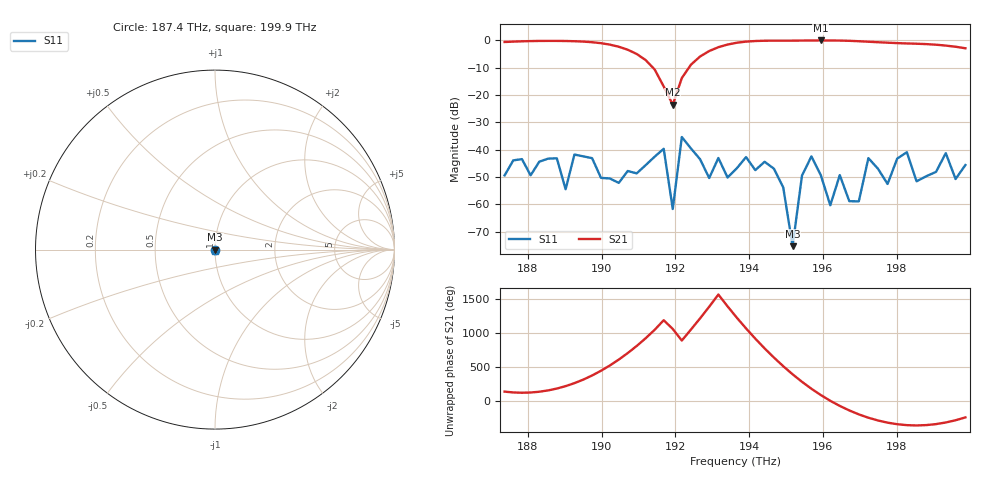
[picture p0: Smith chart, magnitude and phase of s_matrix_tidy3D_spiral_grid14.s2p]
[Version] 2.0
# Hz S RI
[Number of Ports] 2
[Two-Port Data Order] 12_21
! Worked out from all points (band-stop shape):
!   51 points, 187.4 THz to 199.9 THz, reference 50 ohm
!   highest |S21| = -0.05 dB at 195.9 THz (marker M1); lowest = -23.5 dB at 191.9 THz (marker M2)
!   |S21| within 3 dB of the highest: start of sweep to 190.6 THz; 193.1 THz to end of sweep
!   lowest |S11| = -75.3 dB at 195.2 THz (marker M3), VSWR 1.00, Z = 50 + j0.0138 ohm
!   |S11| at or under -10 dB: start of sweep to end of sweep
!   S12 and S22 are empty: the file has one direction only
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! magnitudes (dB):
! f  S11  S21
! 187.4 THz  -49.4  -0.6
! 188.8 THz  -43.1  -0.2
! 189 THz  -54.5  -0.3
! 189.5 THz  -42.4  -0.5
! 190.5 THz  -52.1  -2.3
! 191.7 THz  -39.7  -16.9
! 191.9 THz  -61.7  -23.5
! 192.2 THz  -35.4  -13.8
! 192.9 THz  -50.4  -3.9
! 193.7 THz  -46.8  -0.9
! 194.7 THz  -46.9  -0.1
! 195.2 THz  -75.3  -0.1
! 195.4 THz  -49.5  -0.1
! 195.9 THz  -49.4  -0.1
! 196.2 THz  -60.3  -0.1
! 196.5 THz  -49.3  -0.1
! 197 THz  -58.9  -0.3
! 197.2 THz  -43.1  -0.5
! 197.8 THz  -52.5  -0.9
! 198 THz  -43.2  -1.0
! 198.5 THz  -51.6  -1.2
! 199.9 THz  -45.6  -2.9
